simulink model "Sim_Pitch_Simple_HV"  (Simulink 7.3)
settings: Solver=ode23s  StartTime=0.0  StopTime=200  RelTol=1e-3
InitFcn:
  | init
StartFcn:
  | init
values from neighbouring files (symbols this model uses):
  r2d = 180/pi    (= 57.2957795131)    [init.m]    (also in robust.m)
undefined symbols (not defined in the file or in its folder): Apa, Bpa, Cpa, Dpa, Kmix, Kq

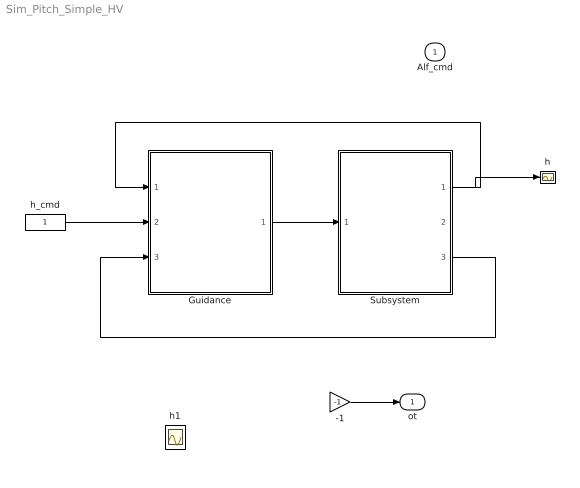
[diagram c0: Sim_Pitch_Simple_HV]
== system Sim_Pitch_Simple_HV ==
  Alf_cmd : Inport  OutDataType=sfix(16)  OutScaling=2^0
  -1 : Gain  Gain=-1  ParameterDataType=sfix(16)  ParameterScaling=2^0  OutDataType=sfix(16)  OutScaling=2^0
  Guidance : Subsystem
  Subsystem : Subsystem
  h : Scope
  h1 : Scope
  h_cmd : Constant  OutDataType=sfix(16)  OutScaling=2^0
  ot : Outport  OutDataType=sfix(16)  OutScaling=2^0
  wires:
  Subsystem/1(h) -> Guidance/1(h), h/1
  h_cmd/1 -> Guidance/2(h_cmd)
  Subsystem/3(hdot) -> Guidance/3(hdot)
  -1/1 -> ot/1
  Guidance/1(Nz_cmd) -> Subsystem/1(Alf_cmd)

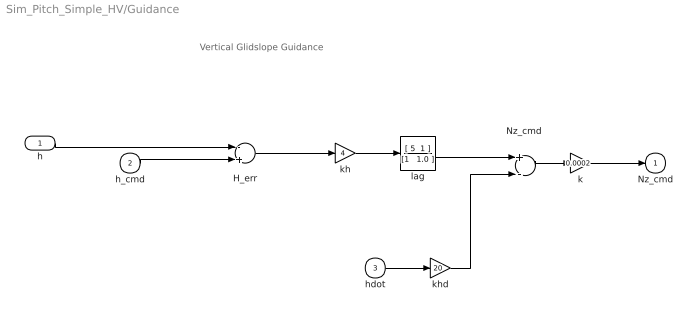
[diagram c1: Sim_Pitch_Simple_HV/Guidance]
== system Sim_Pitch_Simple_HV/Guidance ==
  note: Vertical Glidslope Guidance
  h : Inport  OutDataType=sfix(16)  OutScaling=2^0
  h_cmd : Inport  Port=2  OutDataType=sfix(16)  OutScaling=2^0
  hdot : Inport  Port=3  OutDataType=sfix(16)  OutScaling=2^0
  H_err : Sum  Inputs=-+  OutDataType=sfix(16)  OutScaling=2^0
  "Nz_cmd " : Sum  Inputs=+-  OutDataType=sfix(16)  OutScaling=2^0
  k : Gain  Gain=0.0002  ParameterDataType=sfix(16)  ParameterScaling=2^0  OutDataType=sfix(16)  OutScaling=2^0
  kh : Gain  Gain=4  ParameterDataType=sfix(16)  ParameterScaling=2^0  OutDataType=sfix(16)  OutScaling=2^0
  khd : Gain  Gain=20  ParameterDataType=sfix(16)  ParameterScaling=2^0  OutDataType=sfix(16)  OutScaling=2^0
  lag : TransferFcn  Numerator="[ 5  1 ]"  Denominator="[1   1.0 ]"
  Nz_cmd : Outport  InitialOutput=0
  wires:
  "Nz_cmd "/1 -> k/1
  h/1 -> H_err/1
  H_err/1 -> kh/1
  kh/1 -> lag/1
  k/1 -> Nz_cmd/1
  h_cmd/1 -> H_err/2
  hdot/1 -> khd/1
  khd/1 -> "Nz_cmd "/2
  lag/1 -> "Nz_cmd "/1

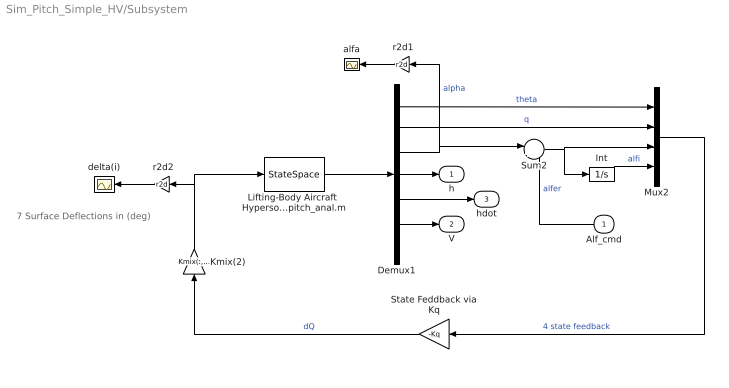
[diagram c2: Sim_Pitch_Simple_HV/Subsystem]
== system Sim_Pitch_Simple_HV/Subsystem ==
  note: 7 Surface Deflections in (deg)
  Alf_cmd : Inport  OutDataType=sfix(16)  OutScaling=2^0
  " r2d1" : Gain  Gain=r2d  ParameterDataType=sfix(16)  ParameterScaling=2^0  OutDataType=sfix(16)  OutScaling=2^0
  " r2d2" : Gain  Gain=r2d  ParameterDataType=sfix(16)  ParameterScaling=2^0  OutDataType=sfix(16)  OutScaling=2^0
  Demux1 : Demux  Outputs=7
  Int : Integrator
  Kmix(2) : Gain  Gain=Kmix(:,2)  Multiplication=Matrix(K*u)  ParameterDataType=sfix(16)  ParameterScaling=2^0  OutDataType=sfix(16)  OutScaling=2^0
  Lifting-Body Aircraft  Hypersonic Pitch  Analysis Model from file pitch_anal.m : StateSpace  A=Apa  B=Bpa  C=Cpa  D=Dpa
  Mux2 : Mux
  State Feddback via Kq : Gain  Gain=-Kq  Multiplication=Matrix(K*u)  ParameterDataType=sfix(16)  ParameterScaling=2^0  OutDataType=sfix(16)  OutScaling=2^0
  Sum2 : Sum  Inputs=|+-  OutDataType=sfix(16)  OutScaling=2^0
  alfa : Scope
  delta(i) : Scope
  h : Outport  OutDataType=sfix(16)  OutScaling=2^0
  V : Outport  Port=2  OutDataType=sfix(16)  OutScaling=2^0
  hdot : Outport  Port=3  OutDataType=sfix(16)  OutScaling=2^0
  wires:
  Mux2/1 -> State Feddback via Kq/1  "4 state feedback"
  State Feddback via Kq/1 -> Kmix(2)/1  "dQ"
  Lifting-Body Aircraft  Hypersonic Pitch  Analysis Model from file pitch_anal.m/1 -> Demux1/1
  " r2d1"/1 -> alfa/1
  Kmix(2)/1 -> Lifting-Body Aircraft  Hypersonic Pitch  Analysis Model from file pitch_anal.m/1, " r2d2"/1
  " r2d2"/1 -> delta(i)/1
  Demux1/1 -> Mux2/1  "theta"
  Demux1/2 -> Mux2/2  "q"
  Int/1 -> Mux2/4  "alfi"
  Demux1/3 -> " r2d1"/1, Sum2/1  "alpha"
  Demux1/6 -> V/1
  Demux1/5 -> hdot/1
  Demux1/4 -> h/1
  Sum2/1 -> Mux2/3, Int/1
  Alf_cmd/1 -> Sum2/2  "alfer"
